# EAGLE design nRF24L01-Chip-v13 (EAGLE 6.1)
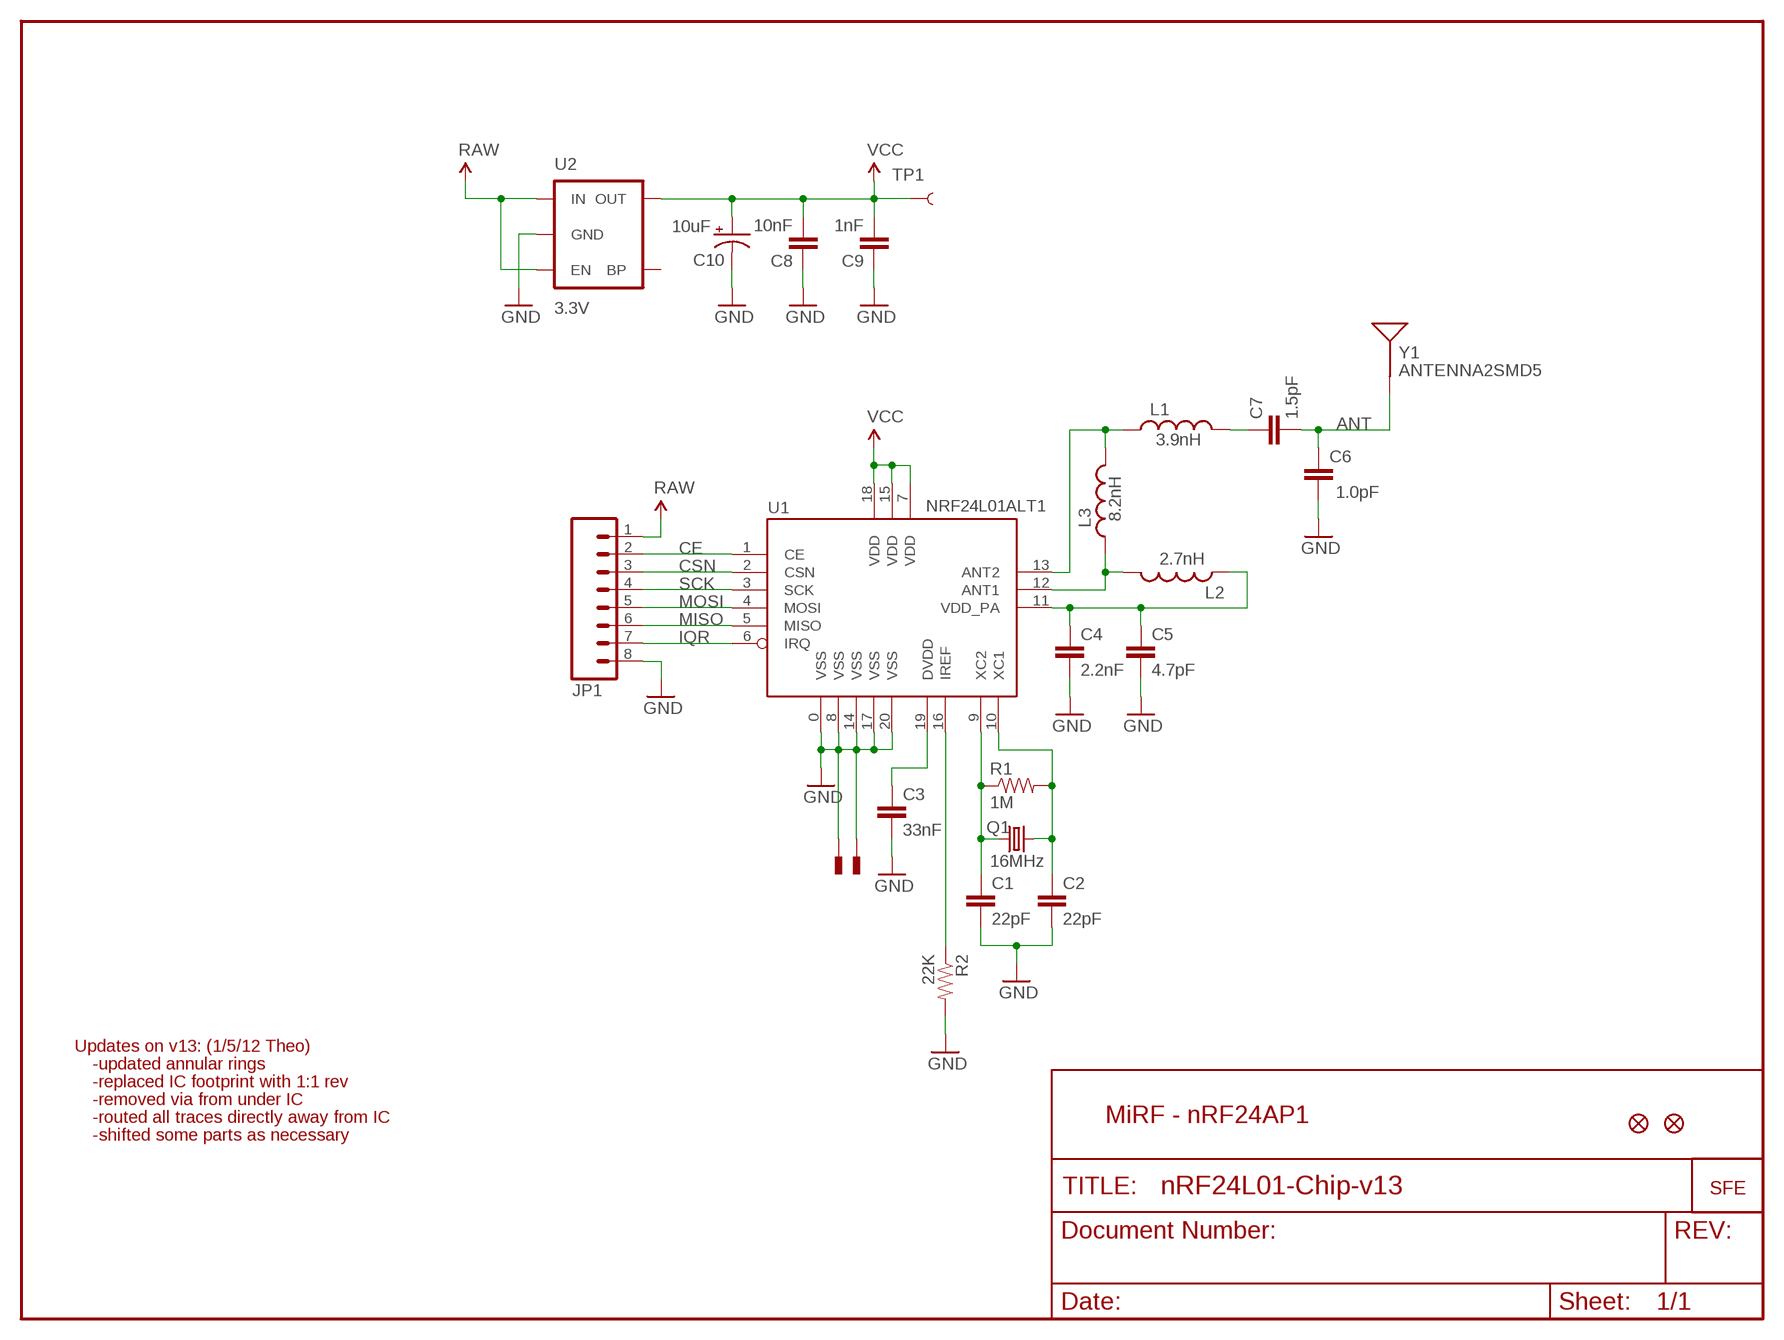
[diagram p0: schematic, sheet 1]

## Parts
C1  22pF  CAP0402-CAP  [0402-CAP]
C2  22pF  CAP0402-CAP  [0402-CAP]
C3  33nF  CAP0402-CAP  [0402-CAP]
C4  2.2nF  CAP0402-CAP  [0402-CAP]
C5  4.7pF  CAP0402-CAP  [0402-CAP]
C6  1.0pF  CAP0402-CAP  [0402-CAP]
C7  1.5pF  CAP0402-CAP  [0402-CAP]
C8  10nF  CAP0402-CAP  [0402-CAP]
C9  1nF  CAP0402-CAP  [0402-CAP]
C10  10uF  CAP_POL1206  [EIA3216]
JP1  M081X08  [1X08]
JP2  FIDUCIALUFIDUCIAL  [MICRO-FIDUCIAL]
JP3  FIDUCIALUFIDUCIAL  [MICRO-FIDUCIAL]
L1  3.9nH  INDUCTOR0402  [C0402]
L2  2.7nH  INDUCTOR0402  [C0402]
L3  8.2nH  INDUCTOR0402  [C0402]
Q1  16MHz  CRYSTAL5X3  [CRYSTAL-SMD-5X3]
R1  1M  RESISTOR0402-RES  [0402-RES]
R2  22K  RESISTOR0402-RES  [0402-RES]
TP1  TEST-POINT3X5  [PAD.03X.05]
U1  NRF24L01ALT1  [QFN20_ALT1]
U2  3.3V  V_REG_LDOSMD  [SOT23-5]
U$1  PAD  [PAD-0.008]
U$4  PAD  [PAD-0.008]
U$5  LOGO-SFENEW  [SFE-NEW-WEBLOGO]
Y1  ANTENNA2SMD5  [ANTENNA-CHIP5]

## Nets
ANT: C6.2 C7.2 Y1.FEED(SIGNAL)
CE: JP1.2 U1.1(CE)
CSN: JP1.3 U1.2(CSN)
GND: C1.2 C2.2 C3.2 C4.2 C5.2 C6.1 C8.1 C9.1 C10.C(-) JP1.8 R2.2 U1.0(VSS) U1.8(VSS) U1.14(VSS) U1.17(VSS) U1.20(VSS) U2.2(GND) U$1.P$1 U$4.P$1
IQR: JP1.7 U1.6(IRQ)
MISO: JP1.6 U1.5(MISO)
MOSI: JP1.5 U1.4(MOSI)
N$1: C1.1 Q1.1 R1.1 U1.9(XC2)
N$2: C2.1 Q1.3 R1.2 U1.10(XC1)
N$3: L2.2 L3.1 U1.12(ANT1)
N$4: R2.1 U1.16(IREF)
N$5: C3.1 U1.19(DVDD)
N$6: L1.1 L3.2 U1.13(ANT2)
N$7: C4.1 C5.1 L2.1 U1.11(VDD_PA)
N$9: C7.1 L1.2
RAW: JP1.1 U2.1(IN) U2.3(EN)
SCK: JP1.4 U1.3(SCK)
VCC: C8.2 C9.2 C10.A(+) TP1.P$1 U1.7(VDD) U1.15(VDD) U1.18(VDD) U2.5(OUT)
Unconnected: U2.4(BP)

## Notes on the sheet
- Updates on v13: (1/5/12 Theo)
- -updated annular rings
- -replaced IC footprint with 1:1 rev
- -removed via from under IC
- -routed all traces directly away from IC | MiRF - nRF24AP1
- -shifted some parts as necessary

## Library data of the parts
C1-C9 = SparkFun:CAP: Capacitor
C10 = SparkFun:CAP_POL: Capacitor Polarized
JP1 = SparkFun:M08: Header 8 Standard 8-pin 0.1" header. Use with straight break away headers (SKU : PRT-00116), right angle break away headers (PRT-00553), swiss pins (PRT-00743), machine pins (PRT-00117), and female headers (PRT-00115).
JP2 JP3 = SparkFun:FIDUCIAL: Fiducial Alignment Points
L1-L3 = SparkFun:INDUCTOR: Inductors
Q1 = SparkFun:CRYSTAL: Crystals
R1 R2 = SparkFun:RESISTOR: Resistor
TP1 = SparkFun:TEST-POINT
U1 = Testing:NRF24L01: 2.4GHz Low Power Transceiver This is the very popular, low cost, very low power RF transceiver from Nordic Semiconductor. Simple SPI interface. SKU: COM-00690
U2 = SparkFun:V_REG_LDO: Voltage Regulator LDO Standard 150mA LDO voltage regulator in SOT-23 layout. Micrel part MIC5205. BP (by-pass) pin is used to lower output noise with 470pF cap.
U$1 U$4 = Testing:PAD
U$5 = SparkFun:LOGO-SFE: Spark Fun Electronics PCB Logo
Y1 = SparkFun:ANTENNA2: Antenna

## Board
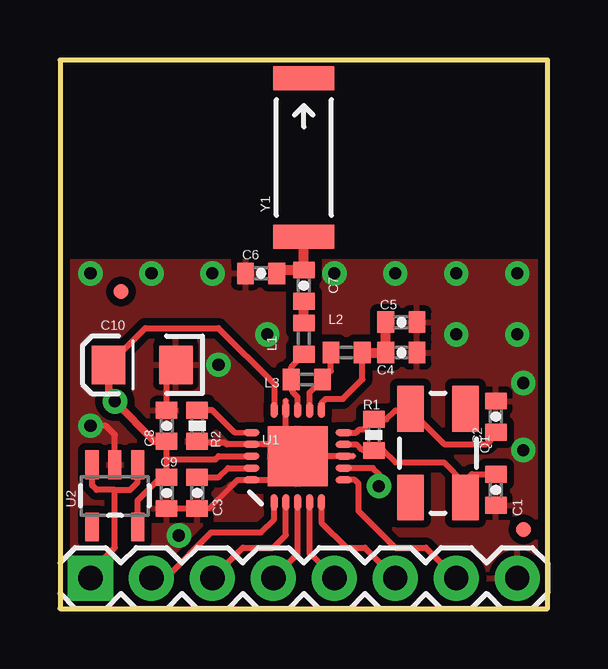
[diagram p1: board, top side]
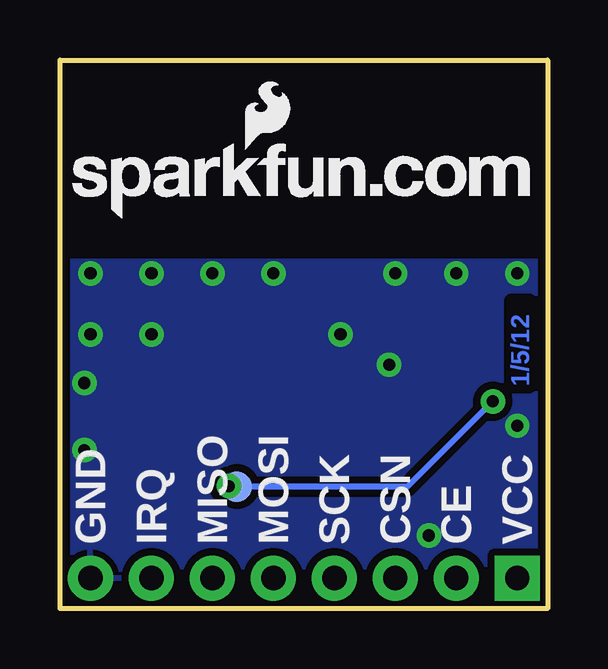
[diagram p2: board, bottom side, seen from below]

Size 20.32 x 22.86 mm. Coordinates in mm from the lower left corner, seen from the top.
Outline: 0,0 20.32,0 20.32,22.86 0,22.86 0,0
Copper layers (1*16): Top 0.035mm / dielectric 1.5mm / Bottom 0.035mm
Design rules: minimum track width 8mil, minimum drill 20mil, track to track 8mil, track to pad 8mil, pad to pad 8mil, via to via 8mil, smd to smd 8mil, copper to edge 8mil, drill to drill 8mil, minimum pad ring 12mil, minimum via ring 10mil, stop-mask expansion 4mil, vias tented up to drill 20mil, thermal gap 10mil
tRestrict: area 7.5,5.1 to 8.4,5.6

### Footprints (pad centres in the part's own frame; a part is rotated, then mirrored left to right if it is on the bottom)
0402-CAP = smd 0.7 x 0.9: 1 -0.65,0; 2 0.65,0
EIA3216 = smd 1.4 x 1.6: A 1.4,0; C -1.4,0
1X08 = drill 1.016 pad 1.88 square: 1 0,0 | drill 1.016 pad 1.88: 2 2.54,0; 3 5.08,0; 4 7.62,0; 5 10.16,0; 6 12.7,0; 7 15.24,0; 8 17.78,0
MICRO-FIDUCIAL = smd 0.635 x 0.635: 1 0,0
C0402 = smd 0.7 x 0.9: 1 -0.65,0; 2 0.65,0
CRYSTAL-SMD-5X3 = smd 1.9 x 1.1: 1 -1.85,-1.15; 2 1.85,-1.15; 3 1.85,1.15; 4 -1.85,1.15
0402-RES = smd 0.7 x 0.9: 1 -0.65,0; 2 0.65,0
PAD.03X.05 = smd 1.27 x 1.27: P$1 0,0
QFN20_ALT1 = smd 2.515 x 2.515: 0 0,0 | smd 0.686 x 0.293: 1 -1.925,0.986; 2 -1.925,0.493; 3 -1.925,0; 4 -1.925,-0.493; 5 -1.925,-0.986; 11 1.925,-0.986; 12 1.925,-0.493; 13 1.925,0; 14 1.925,0.493; 15 1.925,0.986 | smd 0.293 x 0.686: 6 -0.986,-1.925; 7 -0.493,-1.925; 8 0,-1.925; 9 0.493,-1.925; 10 0.986,-1.925; 16 0.986,1.925; 17 0.493,1.925; 18 0,1.925; 19 -0.493,1.925; 20 -0.986,1.925
SOT23-5 = smd 0.55 x 1.2: 1 -0.95,-1.3; 2 0,-1.3; 3 0.95,-1.3; 4 0.95,1.3; 5 -0.95,1.3
PAD-0.008 = smd 0.203 x 0.203: P$1 0,0
ANTENNA-CHIP5 = smd 1.016 x 2.54: FEED -3.302,0; NC 3.302,0

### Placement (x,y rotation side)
C1  18.16,4.95 270 top
C2  18.16,8 90 top
C3  5.71,4.83 270 top
C4  14.22,10.67 0 top
C5  14.22,11.94 0 top
C6  8.38,13.97 0 top
C7  10.16,13.46 90 top
C8  4.45,7.62 270 top
C9  4.45,4.83 90 top
C10  3.43,10.16 180 top
JP1  1.27,1.27 0 top
JP2  2.54,13.21 0 top
JP3  19.3,3.3 0 top
L1  10.16,11.25 90 top
L2  11.94,10.67 180 top
L3  10.29,9.55 180 top
Q1  15.75,6.48 90 top
R1  13.08,7.24 90 top
R2  5.71,7.62 270 top
TP1  12.95,5.08 0 bottom
U1  9.91,6.35 90 top
U2  2.29,4.7 180 top
U$1  9.4,8.66 0 top
U$4  12.22,6.35 0 top
U$5  19.81,16.26 0 bottom
Y1  10.16,18.8 90 top

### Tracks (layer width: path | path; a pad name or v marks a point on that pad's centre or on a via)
ANT
  Top 0.203: C6.2 9.14,13.97 9.28,14.11
  Top 0.406: 9.28,14.11 C7.2 10.16,14.22 Y1.FEED
CE
  Top 0.254: U1.1 8.92,3.71 8.38,3.17 6.3,3.17 4.42,1.29 3.83,1.29 JP1.2
CSN
  Top 0.254: JP1.3 7.62,2.54 8.89,2.54 9.41,3.06 U1.2
GND  (via drill 0.51)
  Top 0.203: C3.2 6.21,4.18 7.11,5.08
  Top 0.254: C10.C 4.45,9.91 C8.1 | C3.2 C9.1 | v1.27,7.62 1.91,7.62 2.29,7.24 U2.2 | 9.41,6.84 U1.17 6.95,6.84 6.88,6.91 5.78,6.91 R2.2 | 9.41,6.84 U1.14 9.41,8.65 U$1.P$1 | 9.41,6.84 U1.0 8.92,5.36 U1.20 7.4,5.36 7.11,5.08 | 10.16,6.35 U$4.P$1 U1.8
  other vias: 4.95,3.05 1.27,13.97 3.81,13.97 6.35,13.97 6.6,10.16 8.64,11.43 11.43,13.97 13.97,13.97 16.51,13.97 19.05,13.97 16.51,11.43 19.05,11.43 19.3,9.4 19.3,6.6
  pour Bottom (isolate 0.305): 0,0 0,14.48 20.32,14.48 20.32,0
  pour Top (isolate 0.305): 0,0 0,14.48 20.32,14.48 20.32,0
IQR
  Top 0.254: JP1.7 15.24,2.54 13.97,2.54 12.45,4.06 12.45,5.21 12.29,5.36 U1.6
MISO
  Top 0.254: JP1.6 12.7,2.54 11.94,2.54 10.89,3.59 U1.5
MOSI
  Top 0.254: U1.4 10.4,2.3 JP1.5
N$1
  Top 0.254: R1.1 13.08,6.6 | R1.1 13.48,6.59 13.97,6.1 16,6.1 16.83,5.27 | 16.83,5.27 16.89,5.21 16.89,4.95 | 16.89,4.95 16.89,4.7 16.9,4.69 Q1.1 | 16.89,4.95 17.02,4.95 17.29,5.22 | 16.83,5.27 16.76,5.21 | C1.1 17.16,5.6 16.83,5.27 | U1.9 12.36,6.84 12.57,6.63 13.04,6.63 R1.1
N$2
  Top 0.254: 14.6,8.38 14.61,8.38 14.61,8.76 | 14.6,8.38 Q1.3 14.6,8.26 16,6.86 17.78,6.86 18.16,7.24 C2.1 | 14.6,8.38 14.48,8.26 13.97,8.26 13.6,7.89 R1.2 12.66,7.47 12.47,7.47 12.34,7.34 U1.10
N$3
  Top 0.254: U1.12 10.4,9.01 L3.1 11.29,9.9 L2.2
N$4
  Top 0.254: U1.16 7.25,7.35 6.33,8.27 R2.1
N$5
  Top 0.254: C3.1 6.62,5.48 7,5.86 U1.19
N$6
  Top 0.254: U1.13 9.9,8.81 9.68,9.04 9.68,9.51 L3.2 9.64,10.08 L1.1
N$7
  Top 0.203: 13.57,10.65 | C4.1 13.57,10.65 | 13.57,10.65
  Top 0.254: L2.1 12.6,10.66 12.6,9.55 11.79,8.74 11.07,8.74 10.89,8.55 U1.11
  Top 0.406: 13.57,10.65 C5.1 | 13.59,10.67 | 13.59,10.67 C4.1 | L2.1 13.59,10.67
N$9
  Top 0.203: C7.1 10.16,12.7
  Top 0.406: L1.2 10.16,12.7
RAW
  Top 0.254: U2.1 3.24,5.27 2.92,4.95 2.29,4.95 | 2.29,4.95 1.52,4.95 1.34,5.14 U2.3 | JP1.1 1.27,1.52 2.29,2.54 2.29,4.95
SCK
  Top 0.254: U1.3 9.9,2.29 JP1.4
VCC  (via drill 0.51)
  Top 0.254: U2.5 3.24,4.51 4.21,5.48 C9.2 4.45,6.22 | U1.18 6.61,6.35 6.48,6.22 4.45,6.22 | 4.45,6.22 4.45,6.99 | C10.A 3.56,11.68 6.6,11.68 8.92,9.37 U1.15 | U1.7 13.04,5.86 13.28,5.61 v13.28,5.11
  Top 0.305: C10.A 2.03,8.89 v2.29,8.64 3.94,6.99 4.45,6.99 C8.2
  Bottom 0.254: v13.28,5.11 13.08,5.08 TP1.P$1 5.84,5.08 v2.29,8.64

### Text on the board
Bottom: 1/5/12
bPlace: VCC | CE | CSN | SCK | MOSI | MISO | IRQ | GND
tValues: DNP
